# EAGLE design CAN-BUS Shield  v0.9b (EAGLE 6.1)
DESCRIPTION: microOBD 200 OBD-II Module; HW_REV: 1.4; PCB_REV: C; PCB_SPEC1: Layer Count: 4; PCB_SPEC2: Size: 1.3" x 0.59"; PCB_SPEC3: Finish Thickness: 0.049" - 0.052"; PCB_SPEC4: Copper Weight: 1oz; TITLE: STM1120
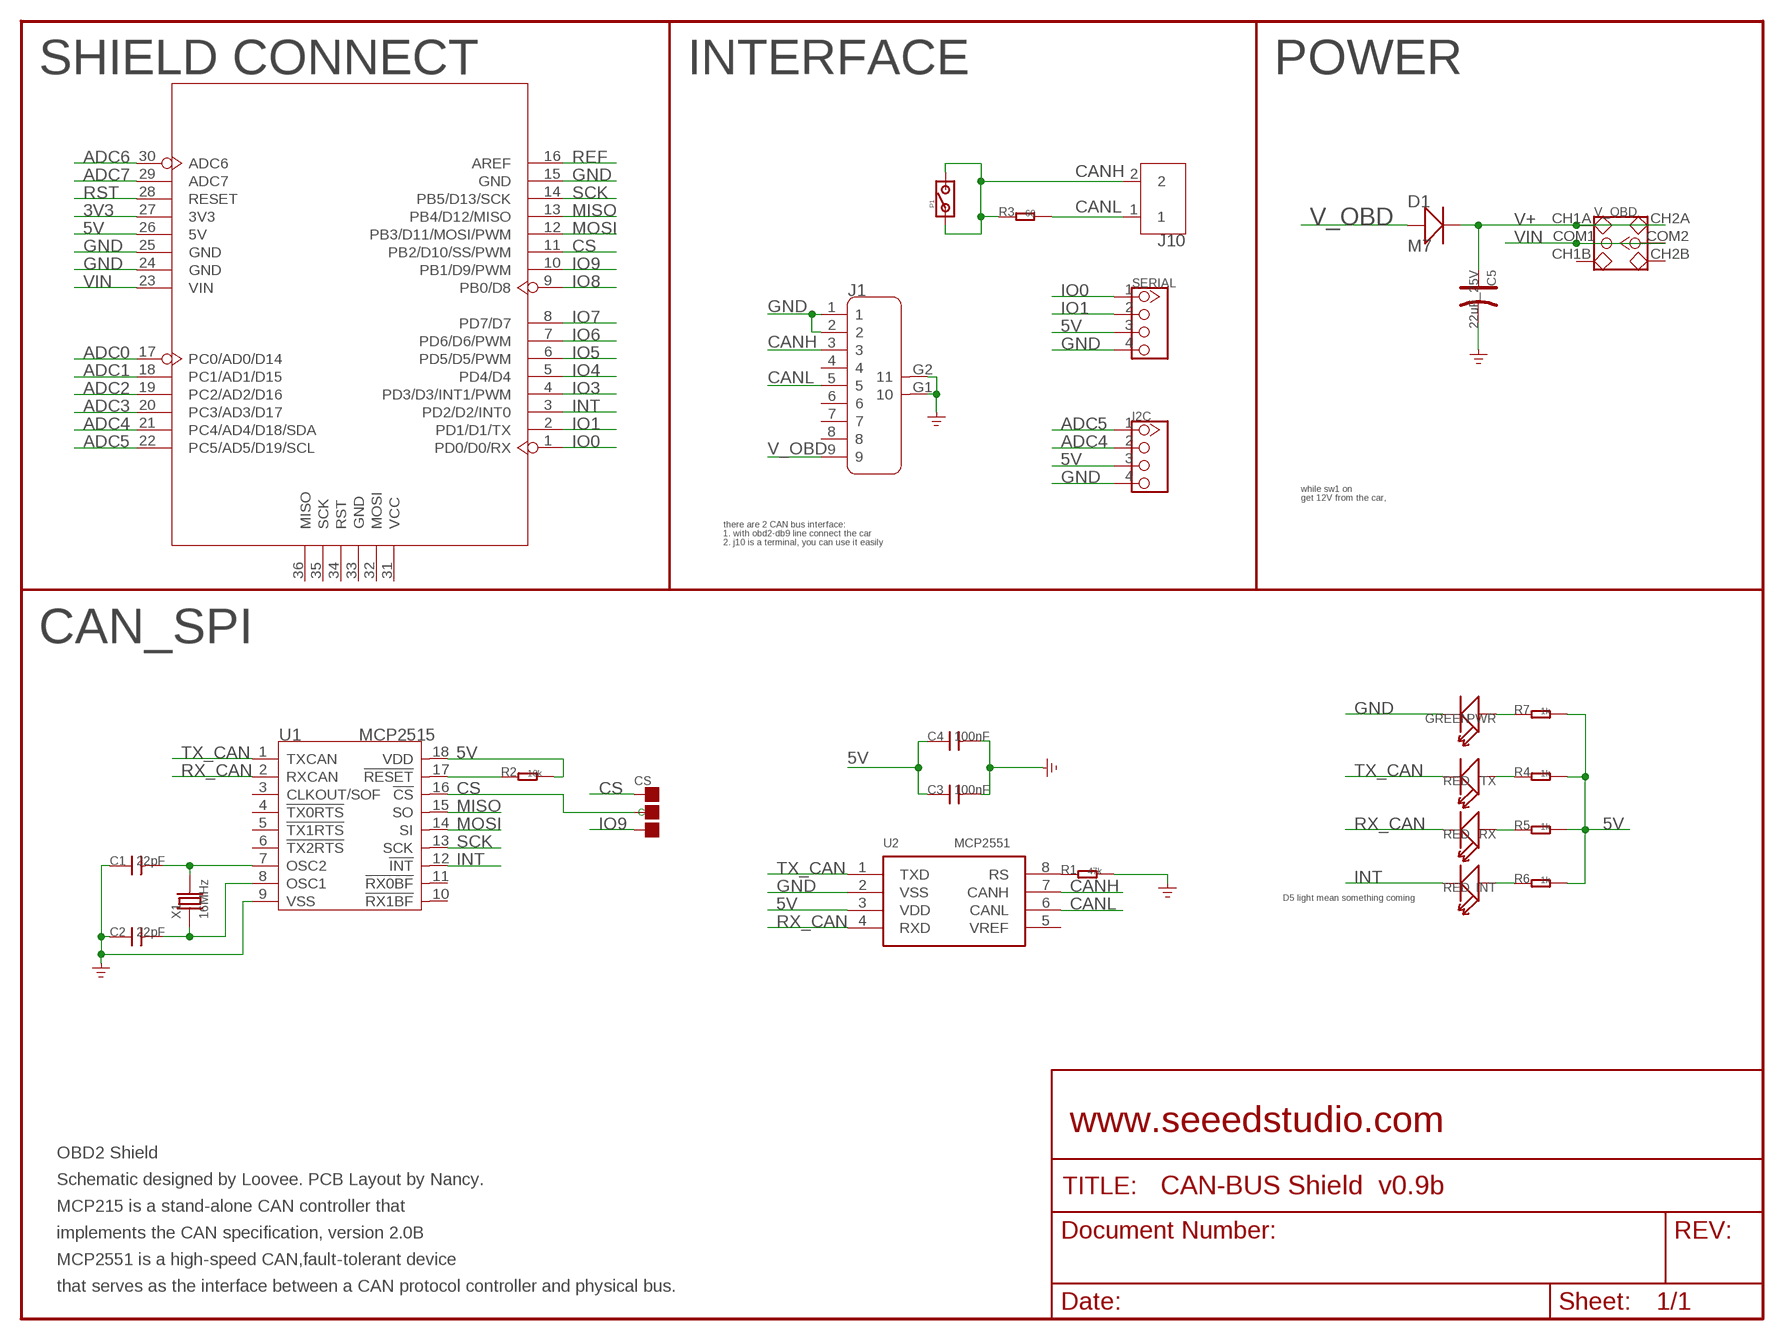
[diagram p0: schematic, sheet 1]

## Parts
C1  22pF  C-0603  [0603]
C2  22pF  C-0603  [0603]
C3  100nF  C-0603  [0603]
C4  100nF  C-0603  [0603]
C5  22uF_25V  CAP-AVX-C  [AVX-C]
CS  PAD-JUMPER-3P-40*40  [3P-SMD-4.1X1.5]
D1  M7  D-SMA  [D2010]
I2C  TWIG-4P-2.0-2.0  [4P-2.0]
INT  RED  LED'0603'  [LED-0603]
J1  DB9'MEAL'  [DB9-MEAL]
J10  SCREW-TERMINAL-2P5.0  [2P-5.0]
P1  PAD-JUMPER-2P  [2P-SMD-1.78X1.27]
PWR  GREEN  LED'0603'  [LED-0603]
R1  47k  R-0603  [0603]
R2  10k  R-0603  [0603]
R3  60  R-0805  [0805]
R4  1k  R-0603  [0603]
R5  1k  R-0603  [0603]
R6  1k  R-0603  [0603]
R7  1k  R-0603  [0603]
RX  RED  LED'0603'  [LED-0603]
SERIAL  TWIG-4P-2.0-2.0  [4P-2.0]
TX  RED  LED'0603'  [LED-0603]
U1  MCP2515  [SOIC18]
U2  MCP2551  [SO08]
U3  ARDUINO  [ARDUINO]
V_OBD  SWITCH-2CH-6P  [6P-2CH-2.54-7.6X3.0]
X1  16MHz  CRYSTAL-HC49S  [HC49/S]

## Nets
3V3: U3.27(3V3)
5V: C3.1 C4.1 I2C.3 R2.2 R4.2 R5.2 R6.2 R7.2 SERIAL.3 U1.18(VDD) U2.3(VDD) U3.26(5V)
ADC0: U3.17(PC0/AD0/D14)
ADC1: U3.18(PC1/AD1/D15)
ADC2: U3.19(PC2/AD2/D16)
ADC3: U3.20(PC3/AD3/D17)
ADC4: I2C.2 U3.21(PC4/AD4/D18/SDA)
ADC5: I2C.1 U3.22(PC5/AD5/D19/SCL)
ADC6: U3.30(ADC6)
ADC7: U3.29(ADC7)
CANH: J1.3 J10.2 P1.1 P1.2 R3.1 U2.7(CANH)
CANL: J1.5 J10.1 R3.2 U2.6(CANL)
CS: CS.00(L) CS.MM(C) U1.16(!CS) U3.11(PB2/D10/SS/PWM)
GND: C1.1 C2.1 C3.2 C4.2 C5.- I2C.4 J1.1 J1.2 J1.G1 J1.G2 PWR.- R1.2 SERIAL.4 U1.9(VSS) U2.2(VSS) U3.15(GND) U3.24(GND) U3.25(GND)
INT: INT.- U1.12(!INT) U3.3(PD2/D2/INT0)
IO0: SERIAL.1 U3.1(PD0/D0/RX)
IO1: SERIAL.2 U3.2(PD1/D1/TX)
IO3: U3.4(PD3/D3/INT1/PWM)
IO4: U3.5(PD4/D4)
IO5: U3.6(PD5/D5/PWM)
IO6: U3.7(PD6/D6/PWM)
IO7: U3.8(PD7/D7)
IO8: U3.9(PB0/D8)
IO9: CS.11(R) U3.10(PB1/D9/PWM)
MISO: U1.15(SO) U3.13(PB4/D12/MISO)
MOSI: U1.14(SI) U3.12(PB3/D11/MOSI/PWM)
N$1: PWR.+ R7.1
N$2: R4.1 TX.+
N$15: R5.1 RX.+
N$16: C1.2 U1.7(OSC2) X1.2
N$17: C2.2 U1.8(OSC1) X1.1
N$19: INT.+ R6.1
N$20: R1.1 U2.8(RS)
REF: U3.16(AREF)
RST: U3.28(RESET)
RST_N: R2.1 U1.17(!RESET)
RX_CAN: RX.- U1.2(RXCAN) U2.4(RXD)
SCK: U1.13(SCK) U3.14(PB5/D13/SCK)
TX_CAN: TX.- U1.1(TXCAN) U2.1(TXD)
V+: C5.+ D1.- V_OBD.CH1A V_OBD.CH2A
V_OBD: D1.+ J1.9
VIN: U3.23(VIN) V_OBD.COM1 V_OBD.COM2
Unconnected: J1.4 J1.6 J1.7 J1.8 U1.3(CLKOUT/SOF) U1.4(!TX0RTS) U1.5(!TX1RTS) U1.6(!TX2RTS) U1.10(!RX1BF) U1.11(!RX0BF) U2.5(VREF) U3.31(VCC) U3.32(MOSI) U3.33(GND) U3.34(RST) U3.35(SCK) U3.36(MISO) V_OBD.CH1B V_OBD.CH2B

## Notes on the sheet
- SHIELD CONNECT | INTERFACE | POWER
- while sw1 on
- get 12V from the car,
- there are 2 CAN bus interface:
- 1. with obd2-db9 line connect the car
- 2. j10 is a terminal, you can use it easily
- CAN_SPI
- D5 light mean something coming
- www.seeedstudio.com
- OBD2 Shield
- Schematic designed by Loovee. PCB Layout by Nancy.
- MCP215 is a stand-alone CAN controller that
- implements the CAN specification, version 2.0B
- MCP2551 is a high-speed CAN,fault-tolerant device
- that serves as the interface between a CAN protocol controller and physical bus.

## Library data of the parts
C1-C4 = Discrete:C*: Ceramic Capacitors
C5 = Discrete:CAP*: Electrolytic Capacitors,Tantalum Capacitors and Super Capacitors
CS = Discrete:PAD-JUMPER-3P
D1 = Discrete:D*
I2C SERIAL = Connector:TWIG-4P-2.0
INT PWR RX TX = Discrete:LED*
J1 = Connector:DB9
J10 = Connector:SCREW-TERMINAL-2P
P1 = Discrete:PAD-JUMPER-2P
R1-R7 = Discrete:R*
U1 = IC:MCP2515: Stand-Alone CAN Controller With SPI Interface
U2 = IC:MCP2551: High-Speed CAN Transceiver http://ww1.microchip.com/downloads/en/devicedoc/21667f.pdf
U3 = Module:ARDUINO
V_OBD = Discrete:SWITCH-2CH-6P
X1 = Discrete:CRYSTAL*: CRYSTAL

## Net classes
0 default: width 0.203 mm, drill 0.305 mm, clearance 0.203 mm

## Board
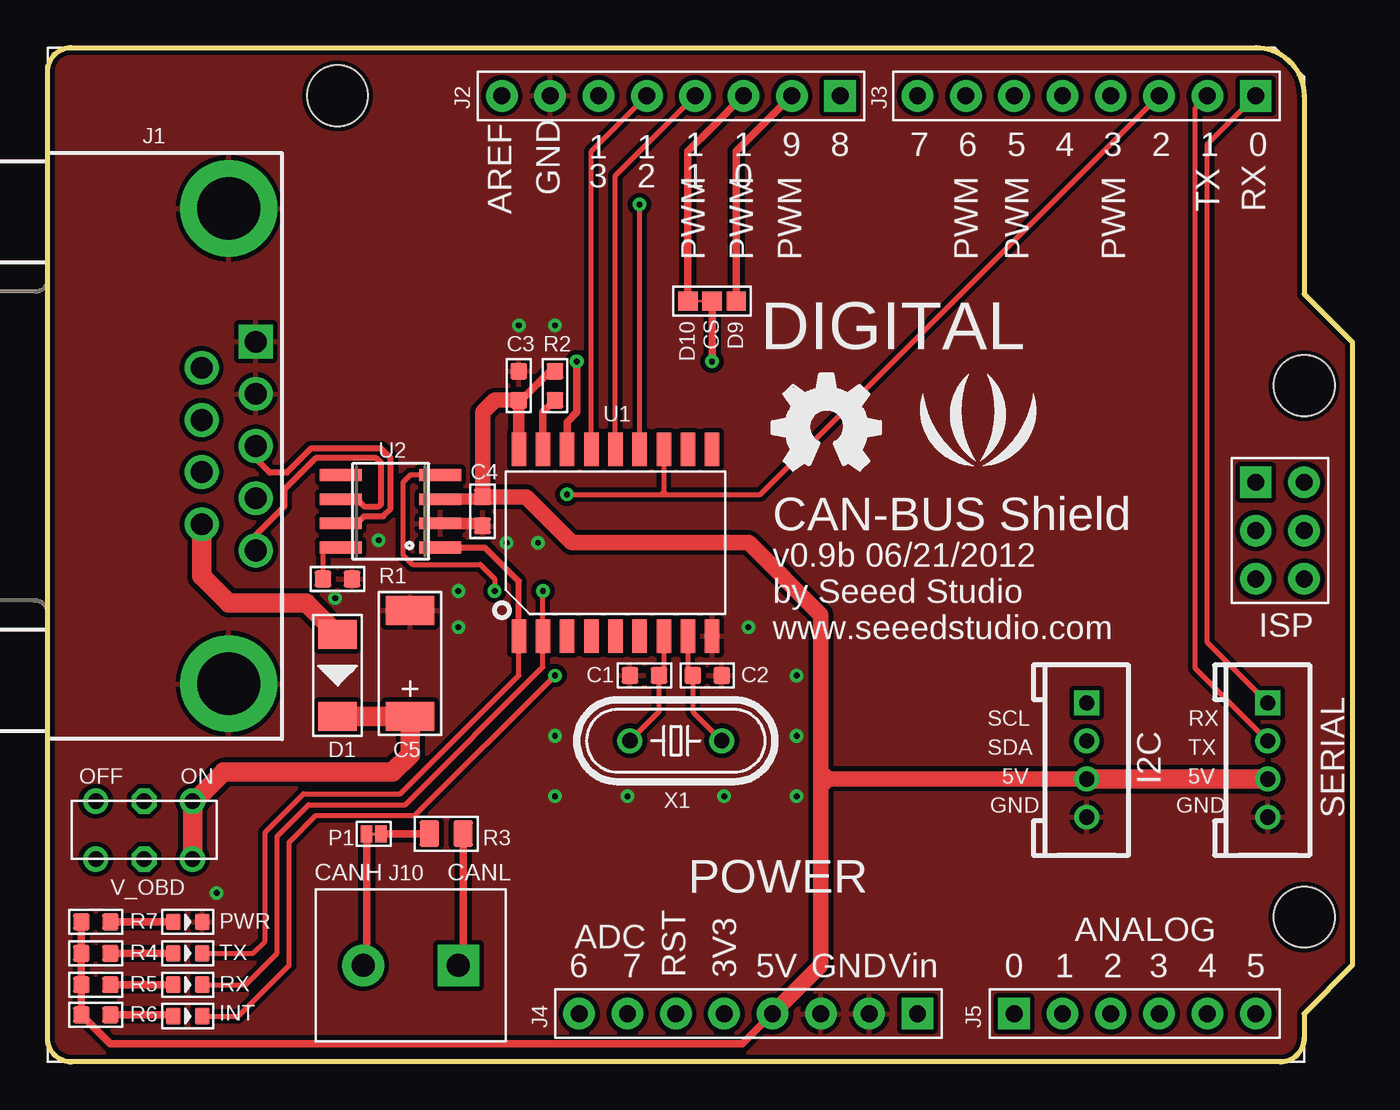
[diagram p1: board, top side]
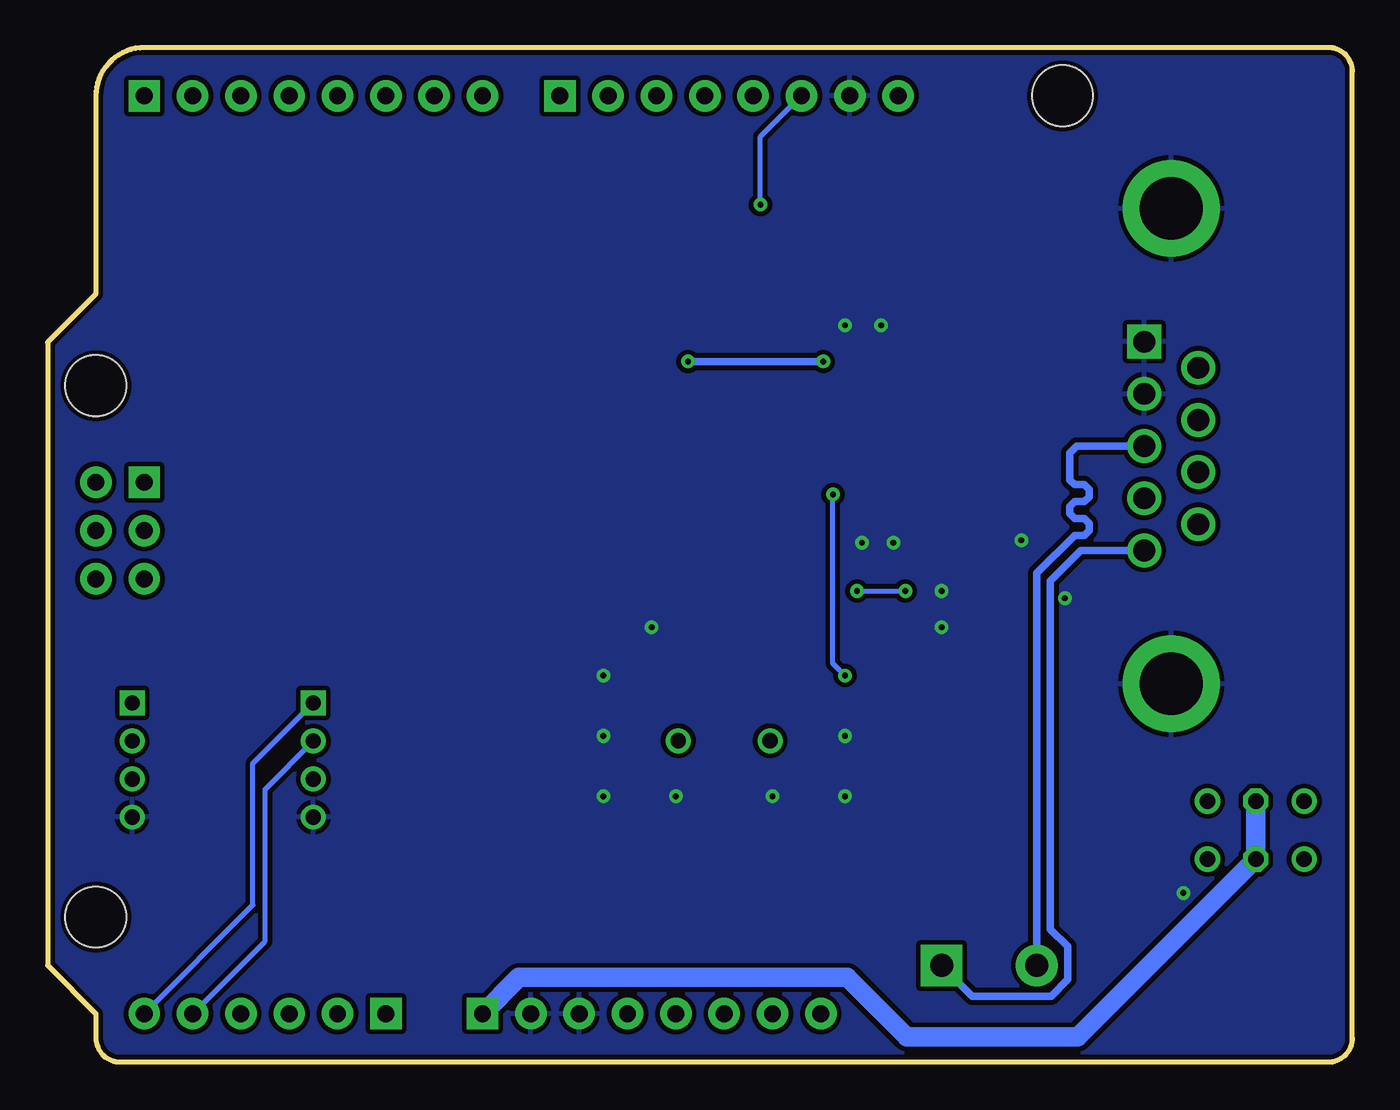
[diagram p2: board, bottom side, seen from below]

Size 68.58 x 53.34 mm. Coordinates in mm from the lower left corner, seen from the top.
Outline: 66.04,2.54 66.04,1.27 arc-90 64.77,0 1.27,0 arc-90 0,1.27 0,52.07 arc-90 1.27,53.34 63.5,53.34 arc-90 66.04,50.8 66.04,40.39 68.58,37.85 68.58,5.08 66.04,2.54
Copper layers (1*16): Top 0.035mm / dielectric 1.5mm / Bottom 0.035mm
Design rules: minimum track width 10mil, minimum drill 12mil, track to track 8mil, track to pad 8mil, pad to pad 8mil, via to via 8mil, smd to smd 8mil, copper to edge 10mil, drill to drill 8mil, minimum pad ring 10mil, minimum via ring 8mil, stop-mask expansion 4mil, vias tented up to drill 25mil, thermal gap 10mil

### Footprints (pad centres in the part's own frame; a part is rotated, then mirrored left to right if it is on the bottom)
0603 = smd 0.889 x 0.889: 1 -0.762,0; 2 0.762,0
AVX-C = smd 1.524 x 2.54: + -2.794,0; - 2.794,0
3P-SMD-4.1X1.5 = smd 1.016 x 1.016: 00 -1.27,0; 11 1.27,0; MM 0,0
D2010 = smd 1.524 x 2.032: + -2.159,0; - 2.159,0
4P-2.0 = drill 0.8 pad 1.27 square: 1 -3,0 | drill 0.8 pad 1.27: 2 -1,0; 3 1,0; 4 3,0
LED-0603 = smd 0.762 x 0.889: + -0.762,0; - 0.762,0
DB9-MEAL = drill 1.143 pad 1.778 square: 1 -5.486,1.422 | drill 1.143 pad 1.778: 2 -2.743,1.422; 3 0,1.422; 4 2.743,1.422; 5 5.486,1.422; 6 -4.115,-1.422; 7 -1.372,-1.422; 8 1.372,-1.422; 9 4.115,-1.422 | drill 3.302 pad 5.08: G1 12.497,0; G2 -12.497,0
2P-5.0 = drill 1.2 pad 2.184 square: 1 0,0 | drill 1.2 pad 2.184: 2 5,0
2P-SMD-1.78X1.27 = smd 0.889 x 0.61: 1 0,0.381; 2 0,-0.381
0805 = smd 1.016 x 1.397: 1 -0.889,0; 2 0.889,0
SOIC18 = smd 0.762 x 1.778: 1 -5.08,-4.915; 2 -3.81,-4.915; 3 -2.54,-4.915; 4 -1.27,-4.915; 5 0,-4.915; 6 1.27,-4.915; 7 2.54,-4.915; 8 3.81,-4.915; 9 5.08,-4.915; 10 5.08,4.915; 11 3.81,4.915; 12 2.54,4.915; 13 1.27,4.915; 14 0,4.915; 15 -1.27,4.915; 16 -2.54,4.915; 17 -3.81,4.915; 18 -5.08,4.915
SO08 = smd 0.61 x 2.21: 1 -1.905,-2.616; 2 -0.635,-2.616; 3 0.635,-2.616; 4 1.905,-2.616; 5 1.905,2.616; 6 0.635,2.616; 7 -0.635,2.616; 8 -1.905,2.616
ARDUINO = drill 0.889 pad 1.651 square: 1 63.5,50.8; 9 41.656,50.8; 17 50.8,2.54; 23 45.72,2.54; 36 63.5,30.48 | drill 0.889 pad 1.651: 2 60.96,50.8; 3 58.42,50.8; 4 55.88,50.8; 5 53.34,50.8; 6 50.8,50.8; 7 48.26,50.8; 8 45.72,50.8; 10 39.116,50.8; 11 36.576,50.8; 12 34.036,50.8; 13 31.496,50.8; 14 28.956,50.8; 15 26.416,50.8; 16 23.876,50.8; 18 53.34,2.54; 19 55.88,2.54; 20 58.42,2.54; 21 60.96,2.54; 22 63.5,2.54; 24 43.18,2.54; 25 40.64,2.54; 26 38.1,2.54; 27 35.56,2.54; 28 33.02,2.54; 29 30.48,2.54; 30 27.94,2.54; 31 66.04,30.48; 32 66.04,27.94; 33 66.04,25.4; 34 63.5,25.4; 35 63.5,27.94 | hole 3.2: 15.24,50.8; 66.04,35.56; 66.04,7.62
6P-2CH-2.54-7.6X3.0 = drill 0.813 pad 1.27: CH1A -1.524,2.54; CH1B -1.524,-2.54; CH2A 1.524,2.54; CH2B 1.524,-2.54 | drill 0.813 pad 1.27 octagon: COM1 -1.524,0; COM2 1.524,0
HC49/S = drill 0.813: 1 -2.413,0; 2 2.413,0

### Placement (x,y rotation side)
C1  31.37,20.32 0 top
C2  34.67,20.32 180 top
C3  24.77,35.56 90 top
C4  22.86,28.96 270 top
C5  19.05,20.95 90 top
CS  34.92,40.01 0 top
D1  15.24,20.32 270 top
I2C  54.61,15.88 270 top
INT  7.37,2.41 0 top
J1  9.53,32.38 270 top
J10  21.59,5.08 180 top
P1  17.14,12 90 top
PWR  7.37,7.37 0 top
R1  15.24,25.4 0 top
R2  26.67,35.56 90 top
R3  20.95,12 0 top
R4  2.54,5.71 180 top
R5  2.54,4.06 180 top
R6  2.54,2.48 180 top
R7  2.54,7.37 180 top
RX  7.37,4.06 0 top
SERIAL  64.14,15.88 270 top
TX  7.37,5.71 0 top
U1  29.84,27.3 0 top
U2  18.03,28.96 90 top
U3  0,0 0 top
U$1  [LOGO_SILK]  48.9,33.02 0 top
U$2  [OSHW_FILLX200_NOTEXT]  38.1,31.11 0 top
V_OBD  5.08,12.19 270 top
X1  33.02,16.89 180 top

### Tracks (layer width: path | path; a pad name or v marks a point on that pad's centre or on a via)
5V
  Top 0.254: R4.2 1.78,5.59
  Top 0.406: 1.78,5.59 R5.2 R6.2 3.3,0.95 36.51,0.95 U3.26 | R4.2 R7.2 | 24.89,34.92 25.02,34.92 26.42,36.32 R2.2
  Top 0.61: U1.18 C3.1 24.89,34.92 | U2.3 21.72,29.59 22.99,29.59 C4.1
  Top 0.813: 40.64,15.24 40.64,23.52 36.85,27.3 27.56,27.3 25.15,29.72 C4.1 22.86,34.16 23.5,34.8 C3.1 | 40.64,15.24 40.64,14.99 | 40.64,14.99 40.64,14.48 | 40.64,14.48 40.64,5.08 U3.26 | I2C.3 41.04,14.88 | 41.01,14.88 40.75,14.88 40.64,14.99 | 41.04,14.88 41.01,14.88 | 41.01,14.88 40.64,15.24 | 41.04,14.88 40.64,14.48
  Top 1.016: I2C.3 SERIAL.3
ADC4
  Bottom 0.254: U3.21 57.15,6.35 57.15,14.34 I2C.2
ADC5
  Bottom 0.254: U3.22 57.78,8.26 57.78,15.7 I2C.1
CANH
  Top 0.152: P1.1 P1.2
  Top 0.305: U2.7 16.26,28.32 16.64,28.7 17.65,28.7 18.03,29.08 18.03,31.75 17.53,32.26 13.84,32.26 12.57,30.99 11.68,30.99 10.95,31.73 J1.3
  Top 0.406: R3.1 P1.2 | P1.1 16.76,5.27 16.59,5.1 J10.2
  Bottom 0.406: J10.2 16.59,25.7 14.61,27.69 14.1,27.69 13.84,27.94 13.84,28.32 14.1,28.57 14.61,28.57 14.86,28.83 14.86,29.21 14.61,29.46 14.1,29.46 13.84,29.72 13.84,30.1 14.1,30.35 14.61,30.35 14.86,30.61 14.86,32.03 14.5,32.38 J1.3 10.92,32.38
CANL
  Top 0.305: U2.6 16.26,29.59 16.64,29.21 17.4,29.21 17.53,29.34 17.53,31.5 17.27,31.75 14.1,31.75 12.45,30.1 12.45,29.21 10.95,27.71 J1.5
  Top 0.406: R3.2 21.84,5.33 J10.1
  Bottom 0.406: J10.1 19.97,3.46 15.84,3.46 14.97,4.34 14.97,6.08 15.88,6.99 15.88,25.3 14.28,26.9 J1.5
CS  (via drill 0.3 pad 0.64)
  Top 0.127: CS.00 CS.MM
  Top 0.406: U3.11 34.92,49.15 33.66,47.88 CS.00 | v34.92,36.83 CS.MM | v27.81,36.83 27.81,34.16 27.3,33.66 U1.16
  Bottom 0.406: v27.81,36.83 v34.92,36.83
GND  (via drill 0.3 pad 0.64)
  Top 0.61: U2.2 22.73,28.32 C4.2
  other vias: 24.13,27.3 17.4,27.43 24.77,38.73 26.67,38.73 25.78,27.3 21.59,22.86 21.59,24.77 15.11,24.38 8.89,8.89 26.67,17.14 26.67,13.97 30.48,13.97 39.37,17.14 39.37,20.32 36.83,22.86 35.56,13.97 39.37,13.97
  pour Top (isolate 0.254): 0,53.34 68.58,53.34 68.58,0 0,0
  pour Bottom (isolate 0.254): 0,53.34 68.58,53.34 68.58,0 0,0
INT  (via drill 0.3 pad 0.64)
  Top 0.254: INT.- 10.03,2.41 12.7,5.08 12.7,11.56 14.1,12.95 19.3,12.95 v26.67,20.32 | U1.12 32.38,29.84 | 32.51,29.84 37.47,29.84 U3.3 | v27.3,29.84 32.26,29.84 | 32.26,29.84 32.38,29.84 | 32.38,29.84 32.51,29.84 | 32.26,29.84 32.38,29.97 32.51,29.84
  Bottom 0.254: v26.67,20.32 27.3,20.95 v27.3,29.84
IO0
  Top 0.254: SERIAL.1 60.96,22.05 60.96,48.26 U3.1
IO1
  Top 0.254: SERIAL.2 60.33,20.68 60.33,50.16 U3.2
IO9
  Top 0.406: CS.11 36.2,47.88 U3.10
MISO
  Top 0.254: U1.15 28.57,47.88 U3.13
MOSI
  Top 0.254: U1.14 29.84,46.61 U3.12
N$1
  Top 0.406: R7.1 PWR.+
N$2
  Top 0.406: R4.1 TX.+
N$15
  Top 0.406: R5.1 RX.+
N$16
  Top 0.254: U1.7 32.38,20.57 C1.2 32.13,18.41 X1.2
N$17
  Top 0.254: U1.8 33.66,20.57 C2.2 33.91,18.41 X1.1
N$19
  Top 0.406: R6.1 6.54,2.48 INT.+
N$20
  Top 0.254: R1.1 14.48,26.8 14.73,27.05 U2.8
RST_N
  Top 0.406: U1.17 26.04,34.16 R2.1
RX_CAN  (via drill 0.3 pad 0.64)
  Top 0.254: RX.- 10.41,4.06 12.06,5.71 12.06,11.87 13.72,13.53 18.8,13.53 26.04,20.77 U1.2 v26.04,24.77 | U2.4 19.05,30.86 18.67,30.48 18.67,26.67 19.18,26.16 22.73,26.16 23.5,25.4 v23.5,24.77
  Bottom 0.254: v26.04,24.77 v23.5,24.77
SCK  (via drill 0.3 pad 0.64)
  Top 0.254: U1.13 31.11,33.27 v31.11,45.09
  Bottom 0.254: v31.11,45.09 31.11,48.64 U3.14
TX_CAN
  Top 0.254: TX.- 10.79,5.71 11.43,6.35 11.43,12.06 13.46,14.1 18.54,14.1 24.77,20.32 U1.1
  Top 0.305: U2.1 22.99,27.05 24.77,25.27 U1.1
V+
  Top 1.016: V_OBD.CH2A V_OBD.CH1A 7.75,13.72 9.27,15.24 18.13,15.24 19.05,16.16 C5.+ D1.-
V_OBD
  Top 1.016: D1.+ 13.59,24.13 9.53,24.13 8.1,25.55 J1.9
VIN
  Bottom 1.016: U3.23 43.81,4.45 26.54,4.45 23.41,1.32 14.43,1.32 V_OBD.COM2 V_OBD.COM1

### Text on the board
tPlace: J2 | J3 | D10 | D9 | CAN-BUS Shield | v0.9b 06/21/2012 | by Seeed Studio | www.seeedstudio.com | SCL | RX | SDA | TX | OFF | ON | 5V | 5V | GND | GND | CANH | CANL | J4 | J5
tNames: ISP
